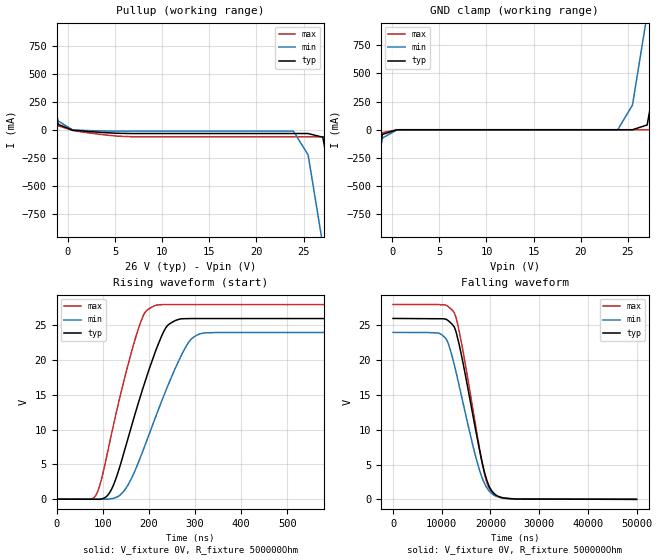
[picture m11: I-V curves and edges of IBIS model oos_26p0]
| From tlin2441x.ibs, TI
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|   oos_26p0 Model
[Model]   oos_26p0
Model_type   Open_source
Polarity   Non-Inverting
Vmeas = 13
Vref = 0
Cref = 2pF
Rref = 500000
|   typ   min   max
C_comp   0.779pF   0.707pF   0.783pF
|  Where Nom  PVT is Nominal Process, 26.0V,   27C
|   Fast PVT is Strong Process,  28.0,   -40C
|   Slow PVT is Weak Process,   24.0V,   150C
[Voltage Range]   26   24   28
|Junction Temperature
[Temperature Range]   27   150   -40
[Pullup Reference]   26   24   28
[Pulldown Reference]   0   0   0
[Power Clamp Reference]   26   24   28
[GND Clamp Reference]   0   0   0
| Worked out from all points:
|   slope of the pullup table from 0 to 3.9 V, typ, clamps not added: 100 ohm
|   falling waveform, V_fixture 0V, R_fixture 500000Ohm: 20-80 % time 4.31us typ, 4.89us min, 4.13us max; typ from 26 V to 0 V
|   rising waveform, V_fixture 0V, R_fixture 500000Ohm: 20-80 % time 72.4ns typ, 85.4ns min, 60.8ns max; typ from 0 V to 26 V
[GND Clamp]
|   Voltage   I(typ)   I(min)   I(max)
-26V      -14.13A    -14.07A    -14.19A
-3.068V   -1.039A    -1.04A     -1.043A
-2.6V     -782.2mA   -785.1mA   -784.7mA
-1.04V    -41.89mA   -74.43mA   -25.95mA
23.92V    2.465nA    2.874nA    2.305nA
25.48V    2.761nA    219.1mA    2.601nA
27.04V    42.7mA     1.027A     2.898nA
28.68V    828.1mA    1.926A     27.32mA
29.61V    1.343A     2.443A     355.2mA
30.78V    1.989A     3.089A     890mA
31.72V    2.507A     3.607A     1.406A
52V       13.8A      14.88A     12.72A
[Pullup]
|   Voltage   I(typ)   I(min)   I(max)
-26V      13.8A      13.77A     13.84A
-3.068V   1.048A     1.047A     1.055A
-2.6V     790mA      790.9mA    796.1mA
-1.04V    47.95mA    78.34mA    36.18mA
520mV     -3.899mA   -1.89mA    -6.989mA
23.92V    -33.78mA   -12.41mA   -62.87mA
25.48V    -33.78mA   -224.2mA   -62.87mA
27.04V    -66.81mA   -1.029A    -62.87mA
28.68V    -840.4mA   -1.925A    -88.38mA
29.61V    -1.354A    -2.441A    -394.5mA
30.78V    -2.001A    -3.091A    -915.7mA
52V       -14.15A    -15.22A    -13.06A
[Ramp]
R_load = 500000
|   typ   min   max
dV/dt_r   15.5958/7.2368e-08   14.392/8.53655e-08   16.7975/6.0818e-08
dV/dt_f   15.5958/4.30782e-06   14.392/4.87396e-06   16.7975/4.13387e-06
[Falling Waveform]
V_fixture = 0V
V_fixture_min = 0V
V_fixture_max = 0V
R_fixture = 500000Ohm
C_fixture = 0F
|   Time   V(typ)   V(min)   V(max)
0s        25.99V     23.99V     28V
9.753us   25.95V     23.77V     27.97V
11.06us   25.81V     22.85V     27.82V
12.56us   24.78V     19.37V     26.83V
14.19us   20.22V     14.43V     21.97V
16.96us   9.97V      6.155V     10.6V
18.68us   4.15V      2.461V     3.967V
19.65us   2.011V     1.286V     1.728V
20.75us   847.6mV    585.3mV    683.7mV
50us      121.7uV    302uV      118.2uV
[Rising Waveform]
V_fixture = 0V
V_fixture_min = 0V
V_fixture_max = 0V
R_fixture = 500000Ohm
C_fixture = 0F
|   Time   V(typ)   V(min)   V(max)
0s        121.6uV    302uV      118.2uV
83.08ns   -9.079mV   -22.74mV   370.8mV
114.7ns   902.1mV    30.52mV    8.052V
145.4ns   6.568V     1.114V     16.88V
180.4ns   14.51V     5.795V     25.13V
196.5ns   17.88V     8.626V     27.2V
232.5ns   24.16V     14.91V     27.98V
290ns     25.97V     22.89V     27.98V
351.1ns   25.98V     23.97V     27.98V
50us      25.99V     23.99V     28V
